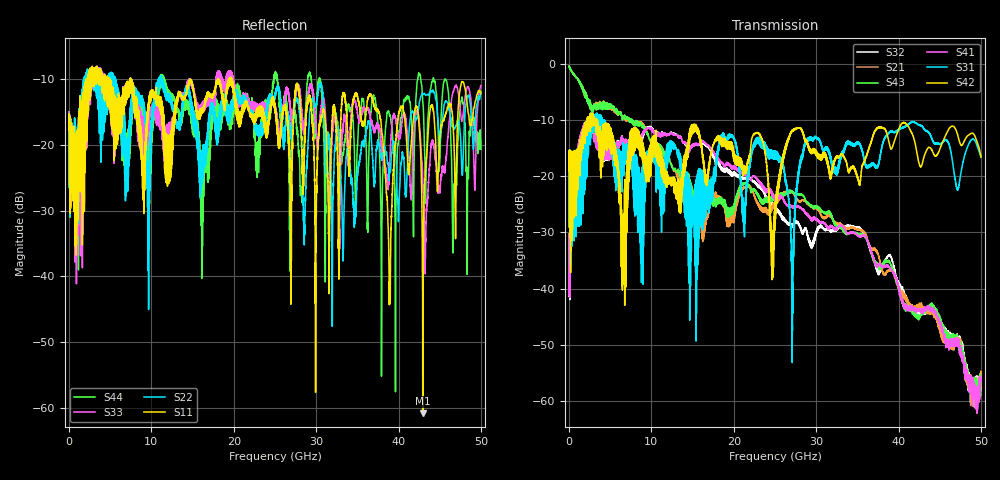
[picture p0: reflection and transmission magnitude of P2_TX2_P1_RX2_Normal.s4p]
!Keysight Technologies,N5225A,MY51441389,A.10.49.11
!Date: Monday, July 08, 2019 13:17:24
!Correction: S11(Full 4 Port(1,2,3,4))
!S12(Full 4 Port(1,2,3,4))
!S13(Full 4 Port(1,2,3,4))
!S14(Full 4 Port(1,2,3,4))
!S21(Full 4 Port(1,2,3,4))
!S22(Full 4 Port(1,2,3,4))
!S23(Full 4 Port(1,2,3,4))
!S24(Full 4 Port(1,2,3,4))
!S31(Full 4 Port(1,2,3,4))
!S32(Full 4 Port(1,2,3,4))
!S33(Full 4 Port(1,2,3,4))
!S34(Full 4 Port(1,2,3,4))
!S41(Full 4 Port(1,2,3,4))
!S42(Full 4 Port(1,2,3,4))
!S43(Full 4 Port(1,2,3,4))
!S44(Full 4 Port(1,2,3,4))
!S4P File: Measurements: <S11,S12,S13,S14>,
!<S21,S22,S23,S24>,
!<S31,S32,S33,S34>,
!<S41,S42,S43,S44>:
# Hz S  dB  R 50
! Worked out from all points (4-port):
!   5000 points, 10 MHz to 50 GHz, reference 50 ohm
!   strongest paths, dB at 10 MHz, 12.51 GHz, 25.01 GHz, 37.51 GHz, 50 GHz:
!     S42: -19.1, -21.0, -28.6, -11.4, -16.6
!     S31: -19.0, -15.0, -15.6, -18.3, -16.5
!     S41: -32.9, -12.3, -24.2, -35.8, -56.1
!     S43: -0.4, -18.3, -24.1, -35.9, -56.8
!     S21: -0.4, -18.2, -25.2, -33.8, -55.3
!     S32: -32.7, -12.3, -25.7, -37.0, -57.3
!   lowest |S11| = -60.8 dB at 42.94 GHz (marker M1), VSWR 1.00, Z = 50 - j0.0909 ohm
!   |S11| at or under -10 dB: 4.921 GHz to 7.419 GHz (2.498 GHz wide, 40.5 % of centre); 7.521 GHz to 18.07 GHz (10.55 GHz wide, 82.4 % of centre); 19.76 GHz to end of sweep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
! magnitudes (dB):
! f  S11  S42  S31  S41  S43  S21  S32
! 10 MHz  -17.7  -19.1  -19.0  -32.9  -0.4  -0.4  -32.7
! 9.8 GHz  -13.0  -18.1  -16.3  -11.4  -13.4  -13.4  -11.2
! 24.68 GHz  -13.2  -38.0  -16.8  -23.1  -23.6  -25.2  -25.0
! 27.12 GHz  -19.6  -11.7  -47.5  -25.6  -22.8  -22.8  -29.1
! 28.98 GHz  -13.6  -14.3  -13.2  -27.0  -24.8  -25.0  -30.9
! 42.94 GHz  -60.8  -17.4  -11.2  -43.8  -44.4  -43.3  -44.1
! 50 GHz  -12.3  -16.6  -16.5  -56.1  -56.8  -55.3  -57.3
